DATA_BLOCK "IMAC_MOTOR1_I/O"
TITLE =
AUTHOR : HOTTENDO
FAMILY : IMAC
VERSION : 0.2


  STRUCT
   MOTOR1_001_ACOM : WORD ;	//MOTOR1 - Instance 001 : 'AUTO' Mode  Command Interface
   MOTOR1_001_ASTAT : WORD ;	//                        'AUTO' Mode  Status Interface
   MOTOR1_001_OSSTAT : WORD ;	//                        OS Status Word
   MOTOR1_001_OSALARM : WORD ;	//                        OS Alarm Word
   MOTOR1_001_OSCOM : WORD ;	//                        OS Command Interface
   MOTOR1_002_ACOM : WORD ;	//MOTOR1 - Instance 002 : 'AUTO' Mode  Command Interface
   MOTOR1_002_ASTAT : WORD ;	//                        'AUTO' Mode  Status Interface
   MOTOR1_002_OSSTAT : WORD ;	//                        OS Status Word
   MOTOR1_002_OSALARM : WORD ;	//                        OS Alarm Word
   MOTOR1_002_OSCOM : WORD ;	//                        OS Command Interface
   MOTOR1_003_ACOM : WORD ;	//MOTOR1 - Instance 003 : 'AUTO' Mode  Command Interface
   MOTOR1_003_ASTAT : WORD ;	//                        'AUTO' Mode  Status Interface
   MOTOR1_003_OSSTAT : WORD ;	//                        OS Status Word
   MOTOR1_003_OSALARM : WORD ;	//                        OS Alarm Word
   MOTOR1_003_OSCOM : WORD ;	//                        OS Command Interface
   MOTOR1_004_ACOM : WORD ;	//MOTOR1 - Instance 004 : 'AUTO' Mode  Command Interface
   MOTOR1_004_ASTAT : WORD ;	//                        'AUTO' Mode  Status Interface
   MOTOR1_004_OSSTAT : WORD ;	//                        OS Status Word
   MOTOR1_004_OSALARM : WORD ;	//                        OS Alarm Word
   MOTOR1_004_OSCOM : WORD ;	//                        OS Command Interface
   MOTOR1_005_ACOM : WORD ;	//MOTOR1 - Instance 005 : 'AUTO' Mode  Command Interface
   MOTOR1_005_ASTAT : WORD ;	//                        'AUTO' Mode  Status Interface
   MOTOR1_005_OSSTAT : WORD ;	//                        OS Status Word
   MOTOR1_005_OSALARM : WORD ;	//                        OS Alarm Word
   MOTOR1_005_OSCOM : WORD ;	//                        OS Command Interface
   MOTOR1_006_ACOM : WORD ;	//MOTOR1 - Instance 006 : 'AUTO' Mode  Command Interface
   MOTOR1_006_ASTAT : WORD ;	//                        'AUTO' Mode  Status Interface
   MOTOR1_006_OSSTAT : WORD ;	//                        OS Status Word
   MOTOR1_006_OSALARM : WORD ;	//                        OS Alarm Word
   MOTOR1_006_OSCOM : WORD ;	//                        OS Command Interface
   MOTOR1_007_ACOM : WORD ;	//MOTOR1 - Instance 007 : 'AUTO' Mode  Command Interface
   MOTOR1_007_ASTAT : WORD ;	//                        'AUTO' Mode  Status Interface
   MOTOR1_007_OSSTAT : WORD ;	//                        OS Status Word
   MOTOR1_007_OSALARM : WORD ;	//                        OS Alarm Word
   MOTOR1_007_OSCOM : WORD ;	//                        OS Command Interface
   MOTOR1_008_ACOM : WORD ;	//MOTOR1 - Instance 008 : 'AUTO' Mode  Command Interface
   MOTOR1_008_ASTAT : WORD ;	//                        'AUTO' Mode  Status Interface
   MOTOR1_008_OSSTAT : WORD ;	//                        OS Status Word
   MOTOR1_008_OSALARM : WORD ;	//                        OS Alarm Word
   MOTOR1_008_OSCOM : WORD ;	//                        OS Command Interface
   MOTOR1_009_ACOM : WORD ;	//MOTOR1 - Instance 009 : 'AUTO' Mode  Command Interface
   MOTOR1_009_ASTAT : WORD ;	//                        'AUTO' Mode  Status Interface
   MOTOR1_009_OSSTAT : WORD ;	//                        OS Status Word
   MOTOR1_009_OSALARM : WORD ;	//                        OS Alarm Word
   MOTOR1_009_OSCOM : WORD ;	//                        OS Command Interface
   MOTOR1_010_ACOM : WORD ;	//MOTOR1 - Instance 010 : 'AUTO' Mode  Command Interface
   MOTOR1_010_ASTAT : WORD ;	//                        'AUTO' Mode  Status Interface
   MOTOR1_010_OSSTAT : WORD ;	//                        OS Status Word
   MOTOR1_010_OSALARM : WORD ;	//                        OS Alarm Word
   MOTOR1_010_OSCOM : WORD ;	//                        OS Command Interface
   MOTOR1_011_ACOM : WORD ;	//MOTOR1 - Instance 011 : 'AUTO' Mode  Command Interface
   MOTOR1_011_ASTAT : WORD ;	//                        'AUTO' Mode  Status Interface
   MOTOR1_011_OSSTAT : WORD ;	//                        OS Status Word
   MOTOR1_011_OSALARM : WORD ;	//                        OS Alarm Word
   MOTOR1_011_OSCOM : WORD ;	//                        OS Command Interface
   MOTOR1_012_ACOM : WORD ;	//MOTOR1 - Instance 012 : 'AUTO' Mode  Command Interface
   MOTOR1_012_ASTAT : WORD ;	//                        'AUTO' Mode  Status Interface
   MOTOR1_012_OSSTAT : WORD ;	//                        OS Status Word
   MOTOR1_012_OSALARM : WORD ;	//                        OS Alarm Word
   MOTOR1_012_OSCOM : WORD ;	//                        OS Command Interface
   MOTOR1_013_ACOM : WORD ;	//MOTOR1 - Instance 013 : 'AUTO' Mode  Command Interface
   MOTOR1_013_ASTAT : WORD ;	//                        'AUTO' Mode  Status Interface
   MOTOR1_013_OSSTAT : WORD ;	//                        OS Status Word
   MOTOR1_013_OSALARM : WORD ;	//                        OS Alarm Word
   MOTOR1_013_OSCOM : WORD ;	//                        OS Command Interface
   MOTOR1_014_ACOM : WORD ;	//MOTOR1 - Instance 014 : 'AUTO' Mode  Command Interface
   MOTOR1_014_ASTAT : WORD ;	//                        'AUTO' Mode  Status Interface
   MOTOR1_014_OSSTAT : WORD ;	//                        OS Status Word
   MOTOR1_014_OSALARM : WORD ;	//                        OS Alarm Word
   MOTOR1_014_OSCOM : WORD ;	//                        OS Command Interface
   MOTOR1_015_ACOM : WORD ;	//MOTOR1 - Instance 015 : 'AUTO' Mode  Command Interface
   MOTOR1_015_ASTAT : WORD ;	//                        'AUTO' Mode  Status Interface
   MOTOR1_015_OSSTAT : WORD ;	//                        OS Status Word
   MOTOR1_015_OSALARM : WORD ;	//                        OS Alarm Word
   MOTOR1_015_OSCOM : WORD ;	//                        OS Command Interface
   MOTOR1_016_ACOM : WORD ;	//MOTOR1 - Instance 016 : 'AUTO' Mode  Command Interface
   MOTOR1_016_ASTAT : WORD ;	//                        'AUTO' Mode  Status Interface
   MOTOR1_016_OSSTAT : WORD ;	//                        OS Status Word
   MOTOR1_016_OSALARM : WORD ;	//                        OS Alarm Word
   MOTOR1_016_OSCOM : WORD ;	//                        OS Command Interface
   MOTOR1_017_ACOM : WORD ;	//MOTOR1 - Instance 017 : 'AUTO' Mode  Command Interface
   MOTOR1_017_ASTAT : WORD ;	//                        'AUTO' Mode  Status Interface
   MOTOR1_017_OSSTAT : WORD ;	//                        OS Status Word
   MOTOR1_017_OSALARM : WORD ;	//                        OS Alarm Word
   MOTOR1_017_OSCOM : WORD ;	//                        OS Command Interface
   MOTOR1_018_ACOM : WORD ;	//MOTOR1 - Instance 018 : 'AUTO' Mode  Command Interface
   MOTOR1_018_ASTAT : WORD ;	//                        'AUTO' Mode  Status Interface
   MOTOR1_018_OSSTAT : WORD ;	//                        OS Status Word
   MOTOR1_018_OSALARM : WORD ;	//                        OS Alarm Word
   MOTOR1_018_OSCOM : WORD ;	//                        OS Command Interface
   MOTOR1_019_ACOM : WORD ;	//MOTOR1 - Instance 019 : 'AUTO' Mode  Command Interface
   MOTOR1_019_ASTAT : WORD ;	//                        'AUTO' Mode  Status Interface
   MOTOR1_019_OSSTAT : WORD ;	//                        OS Status Word
   MOTOR1_019_OSALARM : WORD ;	//                        OS Alarm Word
   MOTOR1_019_OSCOM : WORD ;	//                        OS Command Interface
   MOTOR1_020_ACOM : WORD ;	//MOTOR1 - Instance 020 : 'AUTO' Mode  Command Interface
   MOTOR1_020_ASTAT : WORD ;	//                        'AUTO' Mode  Status Interface
   MOTOR1_020_OSSTAT : WORD ;	//                        OS Status Word
   MOTOR1_020_OSALARM : WORD ;	//                        OS Alarm Word
   MOTOR1_020_OSCOM : WORD ;	//                        OS Command Interface
   MOTOR1_021_ACOM : WORD ;	//MOTOR1 - Instance 021 : 'AUTO' Mode  Command Interface
   MOTOR1_021_ASTAT : WORD ;	//                        'AUTO' Mode  Status Interface
   MOTOR1_021_OSSTAT : WORD ;	//                        OS Status Word
   MOTOR1_021_OSALARM : WORD ;	//                        OS Alarm Word
   MOTOR1_021_OSCOM : WORD ;	//                        OS Command Interface
   MOTOR1_022_ACOM : WORD ;	//MOTOR1 - Instance 022 : 'AUTO' Mode  Command Interface
   MOTOR1_022_ASTAT : WORD ;	//                        'AUTO' Mode  Status Interface
   MOTOR1_022_OSSTAT : WORD ;	//                        OS Status Word
   MOTOR1_022_OSALARM : WORD ;	//                        OS Alarm Word
   MOTOR1_022_OSCOM : WORD ;	//                        OS Command Interface
   MOTOR1_023_ACOM : WORD ;	//MOTOR1 - Instance 023 : 'AUTO' Mode  Command Interface
   MOTOR1_023_ASTAT : WORD ;	//                        'AUTO' Mode  Status Interface
   MOTOR1_023_OSSTAT : WORD ;	//                        OS Status Word
   MOTOR1_023_OSALARM : WORD ;	//                        OS Alarm Word
   MOTOR1_023_OSCOM : WORD ;	//                        OS Command Interface
   MOTOR1_024_ACOM : WORD ;	//MOTOR1 - Instance 024 : 'AUTO' Mode  Command Interface
   MOTOR1_024_ASTAT : WORD ;	//                        'AUTO' Mode  Status Interface
   MOTOR1_024_OSSTAT : WORD ;	//                        OS Status Word
   MOTOR1_024_OSALARM : WORD ;	//                        OS Alarm Word
   MOTOR1_024_OSCOM : WORD ;	//                        OS Command Interface
   MOTOR1_025_ACOM : WORD ;	//MOTOR1 - Instance 025 : 'AUTO' Mode  Command Interface
   MOTOR1_025_ASTAT : WORD ;	//                        'AUTO' Mode  Status Interface
   MOTOR1_025_OSSTAT : WORD ;	//                        OS Status Word
   MOTOR1_025_OSALARM : WORD ;	//                        OS Alarm Word
   MOTOR1_025_OSCOM : WORD ;	//                        OS Command Interface
   MOTOR1_026_ACOM : WORD ;	//MOTOR1 - Instance 026 : 'AUTO' Mode  Command Interface
   MOTOR1_026_ASTAT : WORD ;	//                        'AUTO' Mode  Status Interface
   MOTOR1_026_OSSTAT : WORD ;	//                        OS Status Word
   MOTOR1_026_OSALARM : WORD ;	//                        OS Alarm Word
   MOTOR1_026_OSCOM : WORD ;	//                        OS Command Interface
   MOTOR1_027_ACOM : WORD ;	//MOTOR1 - Instance 027 : 'AUTO' Mode  Command Interface
   MOTOR1_027_ASTAT : WORD ;	//                        'AUTO' Mode  Status Interface
   MOTOR1_027_OSSTAT : WORD ;	//                        OS Status Word
   MOTOR1_027_OSALARM : WORD ;	//                        OS Alarm Word
   MOTOR1_027_OSCOM : WORD ;	//                        OS Command Interface
   MOTOR1_028_ACOM : WORD ;	//MOTOR1 - Instance 028 : 'AUTO' Mode  Command Interface
   MOTOR1_028_ASTAT : WORD ;	//                        'AUTO' Mode  Status Interface
   MOTOR1_028_OSSTAT : WORD ;	//                        OS Status Word
   MOTOR1_028_OSALARM : WORD ;	//                        OS Alarm Word
   MOTOR1_028_OSCOM : WORD ;	//                        OS Command Interface
   MOTOR1_029_ACOM : WORD ;	//MOTOR1 - Instance 029 : 'AUTO' Mode  Command Interface
   MOTOR1_029_ASTAT : WORD ;	//                        'AUTO' Mode  Status Interface
   MOTOR1_029_OSSTAT : WORD ;	//                        OS Status Word
   MOTOR1_029_OSALARM : WORD ;	//                        OS Alarm Word
   MOTOR1_029_OSCOM : WORD ;	//                        OS Command Interface
   MOTOR1_030_ACOM : WORD ;	//MOTOR1 - Instance 030 : 'AUTO' Mode  Command Interface
   MOTOR1_030_ASTAT : WORD ;	//                        'AUTO' Mode  Status Interface
   MOTOR1_030_OSSTAT : WORD ;	//                        OS Status Word
   MOTOR1_030_OSALARM : WORD ;	//                        OS Alarm Word
   MOTOR1_030_OSCOM : WORD ;	//                        OS Command Interface
   MOTOR1_031_ACOM : WORD ;	//MOTOR1 - Instance 031 : 'AUTO' Mode  Command Interface
   MOTOR1_031_ASTAT : WORD ;	//                        'AUTO' Mode  Status Interface
   MOTOR1_031_OSSTAT : WORD ;	//                        OS Status Word
   MOTOR1_031_OSALARM : WORD ;	//                        OS Alarm Word
   MOTOR1_031_OSCOM : WORD ;	//                        OS Command Interface
   MOTOR1_032_ACOM : WORD ;	//MOTOR1 - Instance 032 : 'AUTO' Mode  Command Interface
   MOTOR1_032_ASTAT : WORD ;	//                        'AUTO' Mode  Status Interface
   MOTOR1_032_OSSTAT : WORD ;	//                        OS Status Word
   MOTOR1_032_OSALARM : WORD ;	//                        OS Alarm Word
   MOTOR1_032_OSCOM : WORD ;	//                        OS Command Interface
   MOTOR1_033_ACOM : WORD ;	//MOTOR1 - Instance 033 : 'AUTO' Mode  Command Interface
   MOTOR1_033_ASTAT : WORD ;	//                        'AUTO' Mode  Status Interface
   MOTOR1_033_OSSTAT : WORD ;	//                        OS Status Word
   MOTOR1_033_OSALARM : WORD ;	//                        OS Alarm Word
   MOTOR1_033_OSCOM : WORD ;	//                        OS Command Interface
   MOTOR1_034_ACOM : WORD ;	//MOTOR1 - Instance 034 : 'AUTO' Mode  Command Interface
   MOTOR1_034_ASTAT : WORD ;	//                        'AUTO' Mode  Status Interface
   MOTOR1_034_OSSTAT : WORD ;	//                        OS Status Word
   MOTOR1_034_OSALARM : WORD ;	//                        OS Alarm Word
   MOTOR1_034_OSCOM : WORD ;	//                        OS Command Interface
   MOTOR1_035_ACOM : WORD ;	//MOTOR1 - Instance 035 : 'AUTO' Mode  Command Interface
   MOTOR1_035_ASTAT : WORD ;	//                        'AUTO' Mode  Status Interface
   MOTOR1_035_OSSTAT : WORD ;	//                        OS Status Word
   MOTOR1_035_OSALARM : WORD ;	//                        OS Alarm Word
   MOTOR1_035_OSCOM : WORD ;	//                        OS Command Interface
   MOTOR1_036_ACOM : WORD ;	//MOTOR1 - Instance 036 : 'AUTO' Mode  Command Interface
   MOTOR1_036_ASTAT : WORD ;	//                        'AUTO' Mode  Status Interface
   MOTOR1_036_OSSTAT : WORD ;	//                        OS Status Word
   MOTOR1_036_OSALARM : WORD ;	//                        OS Alarm Word
   MOTOR1_036_OSCOM : WORD ;	//                        OS Command Interface
   MOTOR1_037_ACOM : WORD ;	//MOTOR1 - Instance 037 : 'AUTO' Mode  Command Interface
   MOTOR1_037_ASTAT : WORD ;	//                        'AUTO' Mode  Status Interface
   MOTOR1_037_OSSTAT : WORD ;	//                        OS Status Word
   MOTOR1_037_OSALARM : WORD ;	//                        OS Alarm Word
   MOTOR1_037_OSCOM : WORD ;	//                        OS Command Interface
   MOTOR1_038_ACOM : WORD ;	//MOTOR1 - Instance 038 : 'AUTO' Mode  Command Interface
   MOTOR1_038_ASTAT : WORD ;	//                        'AUTO' Mode  Status Interface
   MOTOR1_038_OSSTAT : WORD ;	//                        OS Status Word
   MOTOR1_038_OSALARM : WORD ;	//                        OS Alarm Word
   MOTOR1_038_OSCOM : WORD ;	//                        OS Command Interface
   MOTOR1_039_ACOM : WORD ;	//MOTOR1 - Instance 039 : 'AUTO' Mode  Command Interface
   MOTOR1_039_ASTAT : WORD ;	//                        'AUTO' Mode  Status Interface
   MOTOR1_039_OSSTAT : WORD ;	//                        OS Status Word
   MOTOR1_039_OSALARM : WORD ;	//                        OS Alarm Word
   MOTOR1_039_OSCOM : WORD ;	//                        OS Command Interface
   MOTOR1_040_ACOM : WORD ;	//MOTOR1 - Instance 040 : 'AUTO' Mode  Command Interface
   MOTOR1_040_ASTAT : WORD ;	//                        'AUTO' Mode  Status Interface
   MOTOR1_040_OSSTAT : WORD ;	//                        OS Status Word
   MOTOR1_040_OSALARM : WORD ;	//                        OS Alarm Word
   MOTOR1_040_OSCOM : WORD ;	//                        OS Command Interface
   MOTOR1_041_ACOM : WORD ;	//MOTOR1 - Instance 041 : 'AUTO' Mode  Command Interface
   MOTOR1_041_ASTAT : WORD ;	//                        'AUTO' Mode  Status Interface
   MOTOR1_041_OSSTAT : WORD ;	//                        OS Status Word
   MOTOR1_041_OSALARM : WORD ;	//                        OS Alarm Word
   MOTOR1_041_OSCOM : WORD ;	//                        OS Command Interface
   MOTOR1_042_ACOM : WORD ;	//MOTOR1 - Instance 042 : 'AUTO' Mode  Command Interface
   MOTOR1_042_ASTAT : WORD ;	//                        'AUTO' Mode  Status Interface
   MOTOR1_042_OSSTAT : WORD ;	//                        OS Status Word
   MOTOR1_042_OSALARM : WORD ;	//                        OS Alarm Word
   MOTOR1_042_OSCOM : WORD ;	//                        OS Command Interface
   MOTOR1_043_ACOM : WORD ;	//MOTOR1 - Instance 043 : 'AUTO' Mode  Command Interface
   MOTOR1_043_ASTAT : WORD ;	//                        'AUTO' Mode  Status Interface
   MOTOR1_043_OSSTAT : WORD ;	//                        OS Status Word
   MOTOR1_043_OSALARM : WORD ;	//                        OS Alarm Word
   MOTOR1_043_OSCOM : WORD ;	//                        OS Command Interface
   MOTOR1_044_ACOM : WORD ;	//MOTOR1 - Instance 044 : 'AUTO' Mode  Command Interface
   MOTOR1_044_ASTAT : WORD ;	//                        'AUTO' Mode  Status Interface
   MOTOR1_044_OSSTAT : WORD ;	//                        OS Status Word
   MOTOR1_044_OSALARM : WORD ;	//                        OS Alarm Word
   MOTOR1_044_OSCOM : WORD ;	//                        OS Command Interface
   MOTOR1_045_ACOM : WORD ;	//MOTOR1 - Instance 045 : 'AUTO' Mode  Command Interface
   MOTOR1_045_ASTAT : WORD ;	//                        'AUTO' Mode  Status Interface
   MOTOR1_045_OSSTAT : WORD ;	//                        OS Status Word
   MOTOR1_045_OSALARM : WORD ;	//                        OS Alarm Word
   MOTOR1_045_OSCOM : WORD ;	//                        OS Command Interface
   MOTOR1_046_ACOM : WORD ;	//MOTOR1 - Instance 046 : 'AUTO' Mode  Command Interface
   MOTOR1_046_ASTAT : WORD ;	//                        'AUTO' Mode  Status Interface
   MOTOR1_046_OSSTAT : WORD ;	//                        OS Status Word
   MOTOR1_046_OSALARM : WORD ;	//                        OS Alarm Word
   MOTOR1_046_OSCOM : WORD ;	//                        OS Command Interface
   MOTOR1_047_ACOM : WORD ;	//MOTOR1 - Instance 047 : 'AUTO' Mode  Command Interface
   MOTOR1_047_ASTAT : WORD ;	//                        'AUTO' Mode  Status Interface
   MOTOR1_047_OSSTAT : WORD ;	//                        OS Status Word
   MOTOR1_047_OSALARM : WORD ;	//                        OS Alarm Word
   MOTOR1_047_OSCOM : WORD ;	//                        OS Command Interface
   MOTOR1_048_ACOM : WORD ;	//MOTOR1 - Instance 048 : 'AUTO' Mode  Command Interface
   MOTOR1_048_ASTAT : WORD ;	//                        'AUTO' Mode  Status Interface
   MOTOR1_048_OSSTAT : WORD ;	//                        OS Status Word
   MOTOR1_048_OSALARM : WORD ;	//                        OS Alarm Word
   MOTOR1_048_OSCOM : WORD ;	//                        OS Command Interface
   MOTOR1_049_ACOM : WORD ;	//MOTOR1 - Instance 049 : 'AUTO' Mode  Command Interface
   MOTOR1_049_ASTAT : WORD ;	//                        'AUTO' Mode  Status Interface
   MOTOR1_049_OSSTAT : WORD ;	//                        OS Status Word
   MOTOR1_049_OSALARM : WORD ;	//                        OS Alarm Word
   MOTOR1_049_OSCOM : WORD ;	//                        OS Command Interface
   MOTOR1_050_ACOM : WORD ;	//MOTOR1 - Instance 050 : 'AUTO' Mode  Command Interface
   MOTOR1_050_ASTAT : WORD ;	//                        'AUTO' Mode  Status Interface
   MOTOR1_050_OSSTAT : WORD ;	//                        OS Status Word
   MOTOR1_050_OSALARM : WORD ;	//                        OS Alarm Word
   MOTOR1_050_OSCOM : WORD ;	//                        OS Command Interface
  END_STRUCT ;
BEGIN
   MOTOR1_001_ACOM := W#16#0;
   MOTOR1_001_ASTAT := W#16#0;
   MOTOR1_001_OSSTAT := W#16#0;
   MOTOR1_001_OSALARM := W#16#0;
   MOTOR1_001_OSCOM := W#16#0;
   MOTOR1_002_ACOM := W#16#0;
   MOTOR1_002_ASTAT := W#16#0;
   MOTOR1_002_OSSTAT := W#16#0;
   MOTOR1_002_OSALARM := W#16#0;
   MOTOR1_002_OSCOM := W#16#0;
   MOTOR1_003_ACOM := W#16#0;
   MOTOR1_003_ASTAT := W#16#0;
   MOTOR1_003_OSSTAT := W#16#0;
   MOTOR1_003_OSALARM := W#16#0;
   MOTOR1_003_OSCOM := W#16#0;
   MOTOR1_004_ACOM := W#16#0;
   MOTOR1_004_ASTAT := W#16#0;
   MOTOR1_004_OSSTAT := W#16#0;
   MOTOR1_004_OSALARM := W#16#0;
   MOTOR1_004_OSCOM := W#16#0;
   MOTOR1_005_ACOM := W#16#0;
   MOTOR1_005_ASTAT := W#16#0;
   MOTOR1_005_OSSTAT := W#16#0;
   MOTOR1_005_OSALARM := W#16#0;
   MOTOR1_005_OSCOM := W#16#0;
   MOTOR1_006_ACOM := W#16#0;
   MOTOR1_006_ASTAT := W#16#0;
   MOTOR1_006_OSSTAT := W#16#0;
   MOTOR1_006_OSALARM := W#16#0;
   MOTOR1_006_OSCOM := W#16#0;
   MOTOR1_007_ACOM := W#16#0;
   MOTOR1_007_ASTAT := W#16#0;
   MOTOR1_007_OSSTAT := W#16#0;
   MOTOR1_007_OSALARM := W#16#0;
   MOTOR1_007_OSCOM := W#16#0;
   MOTOR1_008_ACOM := W#16#0;
   MOTOR1_008_ASTAT := W#16#0;
   MOTOR1_008_OSSTAT := W#16#0;
   MOTOR1_008_OSALARM := W#16#0;
   MOTOR1_008_OSCOM := W#16#0;
   MOTOR1_009_ACOM := W#16#0;
   MOTOR1_009_ASTAT := W#16#0;
   MOTOR1_009_OSSTAT := W#16#0;
   MOTOR1_009_OSALARM := W#16#0;
   MOTOR1_009_OSCOM := W#16#0;
   MOTOR1_010_ACOM := W#16#0;
   MOTOR1_010_ASTAT := W#16#0;
   MOTOR1_010_OSSTAT := W#16#0;
   MOTOR1_010_OSALARM := W#16#0;
   MOTOR1_010_OSCOM := W#16#0;
   MOTOR1_011_ACOM := W#16#0;
   MOTOR1_011_ASTAT := W#16#0;
   MOTOR1_011_OSSTAT := W#16#0;
   MOTOR1_011_OSALARM := W#16#0;
   MOTOR1_011_OSCOM := W#16#0;
   MOTOR1_012_ACOM := W#16#0;
   MOTOR1_012_ASTAT := W#16#0;
   MOTOR1_012_OSSTAT := W#16#0;
   MOTOR1_012_OSALARM := W#16#0;
   MOTOR1_012_OSCOM := W#16#0;
   MOTOR1_013_ACOM := W#16#0;
   MOTOR1_013_ASTAT := W#16#0;
   MOTOR1_013_OSSTAT := W#16#0;
   MOTOR1_013_OSALARM := W#16#0;
   MOTOR1_013_OSCOM := W#16#0;
   MOTOR1_014_ACOM := W#16#0;
   MOTOR1_014_ASTAT := W#16#0;
   MOTOR1_014_OSSTAT := W#16#0;
   MOTOR1_014_OSALARM := W#16#0;
   MOTOR1_014_OSCOM := W#16#0;
   MOTOR1_015_ACOM := W#16#0;
   MOTOR1_015_ASTAT := W#16#0;
   MOTOR1_015_OSSTAT := W#16#0;
   MOTOR1_015_OSALARM := W#16#0;
   MOTOR1_015_OSCOM := W#16#0;
   MOTOR1_016_ACOM := W#16#0;
   MOTOR1_016_ASTAT := W#16#0;
   MOTOR1_016_OSSTAT := W#16#0;
   MOTOR1_016_OSALARM := W#16#0;
   MOTOR1_016_OSCOM := W#16#0;
   MOTOR1_017_ACOM := W#16#0;
   MOTOR1_017_ASTAT := W#16#0;
   MOTOR1_017_OSSTAT := W#16#0;
   MOTOR1_017_OSALARM := W#16#0;
   MOTOR1_017_OSCOM := W#16#0;
   MOTOR1_018_ACOM := W#16#0;
   MOTOR1_018_ASTAT := W#16#0;
   MOTOR1_018_OSSTAT := W#16#0;
   MOTOR1_018_OSALARM := W#16#0;
   MOTOR1_018_OSCOM := W#16#0;
   MOTOR1_019_ACOM := W#16#0;
   MOTOR1_019_ASTAT := W#16#0;
   MOTOR1_019_OSSTAT := W#16#0;
   MOTOR1_019_OSALARM := W#16#0;
   MOTOR1_019_OSCOM := W#16#0;
   MOTOR1_020_ACOM := W#16#0;
   MOTOR1_020_ASTAT := W#16#0;
   MOTOR1_020_OSSTAT := W#16#0;
   MOTOR1_020_OSALARM := W#16#0;
   MOTOR1_020_OSCOM := W#16#0;
   MOTOR1_021_ACOM := W#16#0;
   MOTOR1_021_ASTAT := W#16#0;
   MOTOR1_021_OSSTAT := W#16#0;
   MOTOR1_021_OSALARM := W#16#0;
   MOTOR1_021_OSCOM := W#16#0;
   MOTOR1_022_ACOM := W#16#0;
   MOTOR1_022_ASTAT := W#16#0;
   MOTOR1_022_OSSTAT := W#16#0;
   MOTOR1_022_OSALARM := W#16#0;
   MOTOR1_022_OSCOM := W#16#0;
   MOTOR1_023_ACOM := W#16#0;
   MOTOR1_023_ASTAT := W#16#0;
   MOTOR1_023_OSSTAT := W#16#0;
   MOTOR1_023_OSALARM := W#16#0;
   MOTOR1_023_OSCOM := W#16#0;
   MOTOR1_024_ACOM := W#16#0;
   MOTOR1_024_ASTAT := W#16#0;
   MOTOR1_024_OSSTAT := W#16#0;
   MOTOR1_024_OSALARM := W#16#0;
   MOTOR1_024_OSCOM := W#16#0;
   MOTOR1_025_ACOM := W#16#0;
   MOTOR1_025_ASTAT := W#16#0;
   MOTOR1_025_OSSTAT := W#16#0;
   MOTOR1_025_OSALARM := W#16#0;
   MOTOR1_025_OSCOM := W#16#0;
   MOTOR1_026_ACOM := W#16#0;
   MOTOR1_026_ASTAT := W#16#0;
   MOTOR1_026_OSSTAT := W#16#0;
   MOTOR1_026_OSALARM := W#16#0;
   MOTOR1_026_OSCOM := W#16#0;
   MOTOR1_027_ACOM := W#16#0;
   MOTOR1_027_ASTAT := W#16#0;
   MOTOR1_027_OSSTAT := W#16#0;
   MOTOR1_027_OSALARM := W#16#0;
   MOTOR1_027_OSCOM := W#16#0;
   MOTOR1_028_ACOM := W#16#0;
   MOTOR1_028_ASTAT := W#16#0;
   MOTOR1_028_OSSTAT := W#16#0;
   MOTOR1_028_OSALARM := W#16#0;
   MOTOR1_028_OSCOM := W#16#0;
   MOTOR1_029_ACOM := W#16#0;
   MOTOR1_029_ASTAT := W#16#0;
   MOTOR1_029_OSSTAT := W#16#0;
   MOTOR1_029_OSALARM := W#16#0;
   MOTOR1_029_OSCOM := W#16#0;
   MOTOR1_030_ACOM := W#16#0;
   MOTOR1_030_ASTAT := W#16#0;
   MOTOR1_030_OSSTAT := W#16#0;
   MOTOR1_030_OSALARM := W#16#0;
   MOTOR1_030_OSCOM := W#16#0;
   MOTOR1_031_ACOM := W#16#0;
   MOTOR1_031_ASTAT := W#16#0;
   MOTOR1_031_OSSTAT := W#16#0;
   MOTOR1_031_OSALARM := W#16#0;
   MOTOR1_031_OSCOM := W#16#0;
   MOTOR1_032_ACOM := W#16#0;
   MOTOR1_032_ASTAT := W#16#0;
   MOTOR1_032_OSSTAT := W#16#0;
   MOTOR1_032_OSALARM := W#16#0;
   MOTOR1_032_OSCOM := W#16#0;
   MOTOR1_033_ACOM := W#16#0;
   MOTOR1_033_ASTAT := W#16#0;
   MOTOR1_033_OSSTAT := W#16#0;
   MOTOR1_033_OSALARM := W#16#0;
   MOTOR1_033_OSCOM := W#16#0;
   MOTOR1_034_ACOM := W#16#0;
   MOTOR1_034_ASTAT := W#16#0;
   MOTOR1_034_OSSTAT := W#16#0;
   MOTOR1_034_OSALARM := W#16#0;
   MOTOR1_034_OSCOM := W#16#0;
   MOTOR1_035_ACOM := W#16#0;
   MOTOR1_035_ASTAT := W#16#0;
   MOTOR1_035_OSSTAT := W#16#0;
   MOTOR1_035_OSALARM := W#16#0;
   MOTOR1_035_OSCOM := W#16#0;
   MOTOR1_036_ACOM := W#16#0;
   MOTOR1_036_ASTAT := W#16#0;
   MOTOR1_036_OSSTAT := W#16#0;
   MOTOR1_036_OSALARM := W#16#0;
   MOTOR1_036_OSCOM := W#16#0;
   MOTOR1_037_ACOM := W#16#0;
   MOTOR1_037_ASTAT := W#16#0;
   MOTOR1_037_OSSTAT := W#16#0;
   MOTOR1_037_OSALARM := W#16#0;
   MOTOR1_037_OSCOM := W#16#0;
   MOTOR1_038_ACOM := W#16#0;
   MOTOR1_038_ASTAT := W#16#0;
   MOTOR1_038_OSSTAT := W#16#0;
   MOTOR1_038_OSALARM := W#16#0;
   MOTOR1_038_OSCOM := W#16#0;
   MOTOR1_039_ACOM := W#16#0;
   MOTOR1_039_ASTAT := W#16#0;
   MOTOR1_039_OSSTAT := W#16#0;
   MOTOR1_039_OSALARM := W#16#0;
   MOTOR1_039_OSCOM := W#16#0;
   MOTOR1_040_ACOM := W#16#0;
   MOTOR1_040_ASTAT := W#16#0;
   MOTOR1_040_OSSTAT := W#16#0;
   MOTOR1_040_OSALARM := W#16#0;
   MOTOR1_040_OSCOM := W#16#0;
   MOTOR1_041_ACOM := W#16#0;
   MOTOR1_041_ASTAT := W#16#0;
   MOTOR1_041_OSSTAT := W#16#0;
   MOTOR1_041_OSALARM := W#16#0;
   MOTOR1_041_OSCOM := W#16#0;
   MOTOR1_042_ACOM := W#16#0;
   MOTOR1_042_ASTAT := W#16#0;
   MOTOR1_042_OSSTAT := W#16#0;
   MOTOR1_042_OSALARM := W#16#0;
   MOTOR1_042_OSCOM := W#16#0;
   MOTOR1_043_ACOM := W#16#0;
   MOTOR1_043_ASTAT := W#16#0;
   MOTOR1_043_OSSTAT := W#16#0;
   MOTOR1_043_OSALARM := W#16#0;
   MOTOR1_043_OSCOM := W#16#0;
   MOTOR1_044_ACOM := W#16#0;
   MOTOR1_044_ASTAT := W#16#0;
   MOTOR1_044_OSSTAT := W#16#0;
   MOTOR1_044_OSALARM := W#16#0;
   MOTOR1_044_OSCOM := W#16#0;
   MOTOR1_045_ACOM := W#16#0;
   MOTOR1_045_ASTAT := W#16#0;
   MOTOR1_045_OSSTAT := W#16#0;
   MOTOR1_045_OSALARM := W#16#0;
   MOTOR1_045_OSCOM := W#16#0;
   MOTOR1_046_ACOM := W#16#0;
   MOTOR1_046_ASTAT := W#16#0;
   MOTOR1_046_OSSTAT := W#16#0;
   MOTOR1_046_OSALARM := W#16#0;
   MOTOR1_046_OSCOM := W#16#0;
   MOTOR1_047_ACOM := W#16#0;
   MOTOR1_047_ASTAT := W#16#0;
   MOTOR1_047_OSSTAT := W#16#0;
   MOTOR1_047_OSALARM := W#16#0;
   MOTOR1_047_OSCOM := W#16#0;
   MOTOR1_048_ACOM := W#16#0;
   MOTOR1_048_ASTAT := W#16#0;
   MOTOR1_048_OSSTAT := W#16#0;
   MOTOR1_048_OSALARM := W#16#0;
   MOTOR1_048_OSCOM := W#16#0;
   MOTOR1_049_ACOM := W#16#0;
   MOTOR1_049_ASTAT := W#16#0;
   MOTOR1_049_OSSTAT := W#16#0;
   MOTOR1_049_OSALARM := W#16#0;
   MOTOR1_049_OSCOM := W#16#0;
   MOTOR1_050_ACOM := W#16#0;
   MOTOR1_050_ASTAT := W#16#0;
   MOTOR1_050_OSSTAT := W#16#0;
   MOTOR1_050_OSALARM := W#16#0;
   MOTOR1_050_OSCOM := W#16#0;
END_DATA_BLOCK

